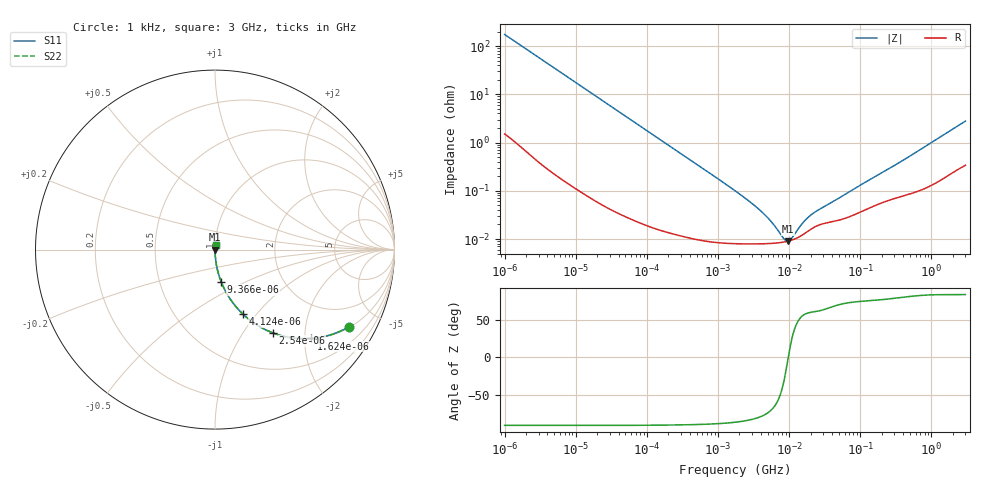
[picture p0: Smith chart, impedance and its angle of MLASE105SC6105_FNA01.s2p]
! MLASE105SC6105_FNA01  S-PARAMETER MODEL  ( Standard Model )
! Model Generated by TAIYO YUDEN Corporation (http://www.ty-top.com)
! Version 1.0
! TAIYO YUDEN Control No. 220601
! Copyright(c) 2012 TAIYO YUDEN CO.,LTD. All Rights Reserved.
! Product Description (link to TY-COMPAS)
! https://ds.yuden.co.jp/TYCOMPAS/or/detail?pn=MLASE105SC6105KFNA01&u=M
! Products Name : Multilayer Ceramic Capacitors
! Characteristics :
!  Capacitance : 1 [uF] , Rated Voltage : 16 [V] , TCC : X6S
!  Case Size : 1.0 x 0.5 / 0.039 x 0.02 [mm/inch] , Thickness : 0.5 / 0.02 [mm/inch]
!  (Conditions: Temperature = 25 [degC] , DC Bias Voltage = 0 [V])
! External Node Assignments :
!  1  o---| |---o  2
! GND o---------o GND
! Frequency Range : 1kHz  -  3GHz  [ 401 STEP ]
# MHZ S RI R 50
! Freq[MHz].  S11 Real  S11 Imag  S21 Real  S21 Imag  S12 Real  S12 Imag  S22 Real  S22 Imag
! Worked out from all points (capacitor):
!   401 points, 1 kHz to 3 GHz, reference 50 ohm
!   read as one part in series: C = 915 nF near 1.077 kHz
!   lowest |Z| = 9 mohm at 9.626 MHz (marker M1)
!   series resonance near 9.708 MHz, so ESL is about 290 pH
!   S11 on the Smith chart (normalised r, x): 1 kHz: 1.03, -3.47; 1.624 kHz: 1.02, -2.15; 2.54 kHz: 1.01, -1.37; 4.124 kHz: 1.01, -0.85; 9.366 kHz: 1.00, -0.37; 3 GHz: 1.01, +0.06
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0.001  0.749 -0.4293  0.251 0.4293  0.251 0.4293  0.749 -0.4293
0.001161  0.69 -0.4582  0.31 0.4582  0.31 0.4582  0.69 -0.4582
0.001624  0.5348 -0.4948  0.4652 0.4948  0.4652 0.4948  0.5348 -0.4948
0.00254  0.322 -0.4637  0.678 0.4637  0.678 0.4637  0.322 -0.4637
0.004124  0.154 -0.3577  0.846 0.3577  0.846 0.3577  0.154 -0.3577
0.005988  0.0802 -0.2685  0.9198 0.2685  0.9198 0.2685  0.0802 -0.2685
0.009366  0.0349 -0.1805  0.9651 0.1805  0.9651 0.1805  0.0349 -0.1805
0.01216  0.0213 -0.1411  0.9787 0.1411  0.9787 0.1411  0.0213 -0.1411
0.033275  0.00317 -0.0527  0.9968 0.0527  0.9968 0.0527  0.00317 -0.0527
0.147855  0.000298 -0.012  0.9997 0.012  0.9997 0.012  0.000298 -0.012
1.732051  8.1e-05 -0.001  0.9999 0.001  0.9999 0.001  8.1e-05 -0.001
3.93371  7.96e-05 -0.000381  0.9999 0.000381  0.9999 0.000381  7.96e-05 -0.000381
5.711239  8.12e-05 -0.000206  0.9999 0.000206  0.9999 0.000206  8.12e-05 -0.000206
7.988506  8.53e-05 -7.3e-05  0.9999 7.3e-05  0.9999 7.3e-05  8.53e-05 -7.3e-05
8.606987  8.69e-05 -4.49e-05  0.9999 4.49e-05  0.9999 4.49e-05  8.69e-05 -4.49e-05
9.625639  9e-05 -3.14e-06  0.9999 3.14e-06  0.9999 3.14e-06  9e-05 -3.14e-06
10.37087  9.27e-05 2.46e-05  0.9999 -2.46e-05  0.9999 -2.46e-05  9.27e-05 2.46e-05
11.1738  9.61e-05 5.25e-05  0.9999 -5.25e-05  0.9999 -5.25e-05  9.61e-05 5.25e-05
15.62917  0.000123 0.000179  0.9999 -0.000179  0.9999 -0.000179  0.000123 0.000179
21.06097  0.000166 0.000286  0.9998 -0.000286  0.9998 -0.000286  0.000166 0.000286
256.0921  0.000645 0.00283  0.9994 -0.00283  0.9994 -0.00283  0.000645 0.00283
3000  0.0041 0.0273  0.9959 -0.0273  0.9959 -0.0273  0.0041 0.0273
